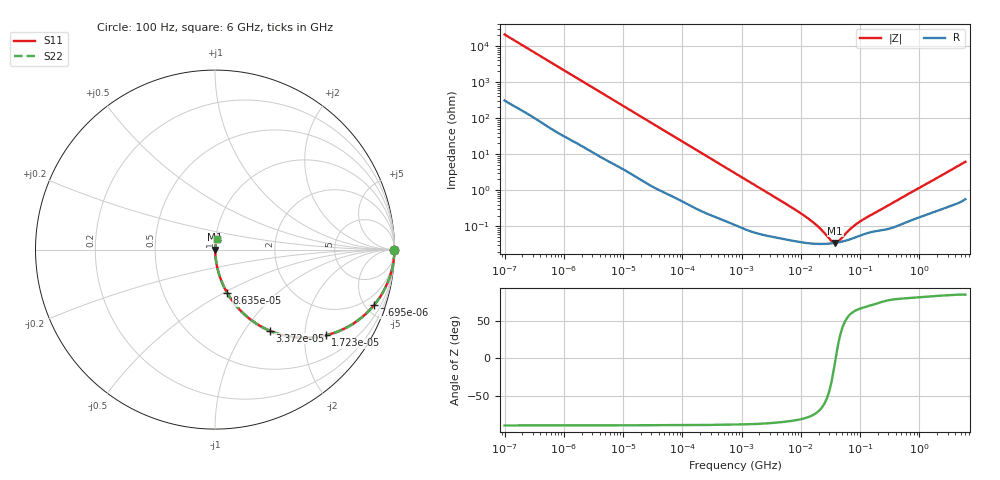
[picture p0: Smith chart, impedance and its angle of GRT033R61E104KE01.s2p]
!Murata Part Number: GRT033R61E104KE01
!These Parameters are Measured in Series Mode Connection
!Data Generated on Jun 19, 2026
!  o--ll--o
!Port1  Port2
!  o------o
!Operation Temp=25[degC], DC Bias Voltage=0[V]
!Freq. Start=100[Hz] Stop=6[GHz] 401[Steps]
# Hz S RI R 50
!Freq.(Hz) S11(Real) S11(Imag) S21(Real) S21(Imag) S12(Real) S12(Imag) S22(Real) S22(Imag)
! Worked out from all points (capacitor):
!   401 points, 100 Hz to 6 GHz, reference 50 ohm
!   read as one part in series: C = 76 nF near 109 Hz
!   lowest |Z| = 34.9 mohm at 38.09 MHz (marker M1)
!   series resonance near 38.76 MHz, so ESL is about 220 pH
!   S11 on the Smith chart (normalised r, x): 100 Hz: open; 7.695 kHz: 1.10, -5.66; 17.23 kHz: 1.04, -2.55; 33.72 kHz: 1.02, -1.31; 86.35 kHz: 1.01, -0.52; 6 GHz: 1.01, +0.12
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100  0.9999 -0.00479  9.37e-05 0.00479  9.37e-05 0.00479  0.9999 -0.00479
627  0.9987 -0.0294  0.0013 0.0294  0.0013 0.0294  0.9987 -0.0294
2008  0.9899 -0.0924  0.0101 0.0924  0.0101 0.0924  0.9899 -0.0924
4496  0.9557 -0.1977  0.0443 0.1977  0.0443 0.1977  0.9557 -0.1977
7695  0.8849 -0.3107  0.1151 0.3107  0.1151 0.3107  0.8849 -0.3107
11514  0.7791 -0.4061  0.2209 0.4061  0.2209 0.4061  0.7791 -0.4061
17227  0.6176 -0.4772  0.3824 0.4772  0.3824 0.4772  0.6176 -0.4772
33721  0.3043 -0.4512  0.6957 0.4512  0.6957 0.4512  0.3043 -0.4512
40335  0.2362 -0.4156  0.7638 0.4156  0.7638 0.4156  0.2362 -0.4156
86348  0.0674 -0.2403  0.9326 0.2403  0.9326 0.2403  0.0674 -0.2403
221108  0.0128 -0.1008  0.9872 0.1008  0.9872 0.1008  0.0128 -0.1008
774597  0.00197 -0.0297  0.998 0.0297  0.998 0.0297  0.00197 -0.0297
6948629  0.000417 -0.00336  0.9996 0.00336  0.9996 0.00336  0.000417 -0.00336
1.555665e7  0.000335 -0.00132  0.9997 0.00132  0.9997 0.00132  0.000335 -0.00132
2.128304e7  0.000327 -0.000804  0.9997 0.000804  0.9997 0.000804  0.000327 -0.000804
3.330331e7  0.000338 -0.000191  0.9997 0.000191  0.9997 0.000191  0.000338 -0.000191
3.80911e7  0.000348 -2.15e-05  0.9997 2.15e-05  0.9997 2.15e-05  0.000348 -2.15e-05
4.35672e7  0.000361 0.000146  0.9996 -0.000146  0.9996 -0.000146  0.000361 0.000146
6.817316e7  0.00044 0.000718  0.9996 -0.000718  0.9996 -0.000718  0.00044 0.000718
9.326766e7  0.000532 0.00115  0.9995 -0.00115  0.9995 -0.00115  0.000532 0.00115
3.124326e8  0.000881 0.00388  0.9991 -0.00388  0.9991 -0.00388  0.000881 0.00388
6e9  0.00931 0.0605  0.9907 -0.0605  0.9907 -0.0605  0.00931 0.0605
